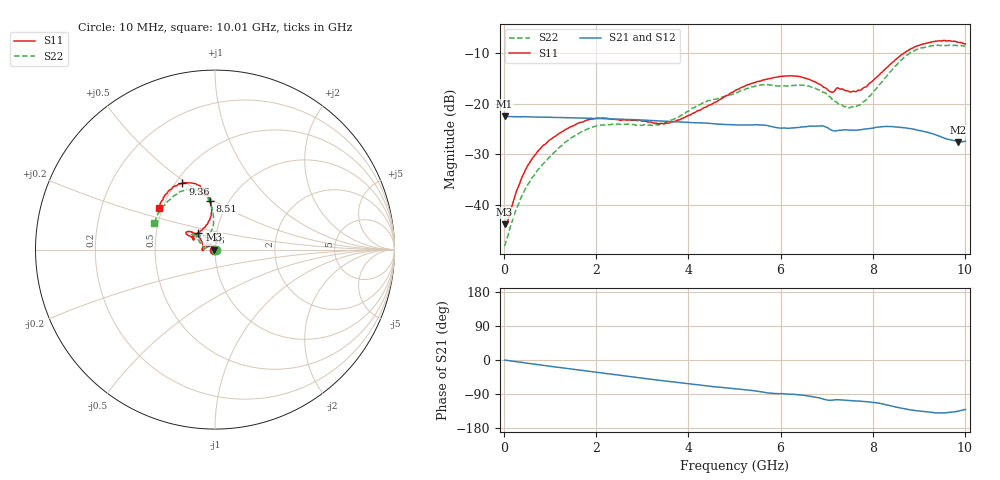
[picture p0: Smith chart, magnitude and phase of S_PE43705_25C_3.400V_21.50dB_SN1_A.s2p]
! Device ID: PE43705
! Serial: 1
! Insertion: A
! Impedance: 50 ohm
! Temp: 25C
! VDD: 3.400V
! Attenuation Step: 21.50dB
#  Hz  S  RI  R  50
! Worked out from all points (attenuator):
!   401 points, 10 MHz to 10.01 GHz, reference 50 ohm
!   highest |S21| = -22.55 dB at 10 MHz (marker M1); lowest = -27.6 dB at 9.86 GHz (marker M2)
!   lowest |S11| = -43.8 dB at 10 MHz (marker M3), VSWR 1.01, Z = 49.4 + j0.0446 ohm
!   |S11| at or under -10 dB: start of sweep to 8.683 GHz
!   |S22| runs from -48.2 to -8.5 dB; largest |S21 - S12| = 0.00085
!   S11 on the Smith chart (normalised r, x): 10 MHz: 0.99, +0.00; 7.46 GHz: 0.81, +0.16; 8.51 GHz: 0.82, +0.48; 9.36 GHz: 0.54, +0.48; 10.01 GHz: 0.48, +0.26
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1e7  -0.00643 0.000452  0.0746 -0.000322  0.0748 -0.000277  0.0039 0.000332
8.5e7  -0.00617 0.00348  0.0744 -0.00196  0.0744 -0.00195  0.00426 0.00266
3.85e8  -0.0101 0.0156  0.0735 -0.00808  0.0738 -0.00812  0.000149 0.0123
6.6e8  -0.0194 0.0236  0.0724 -0.0141  0.0724 -0.014  -0.0085 0.0178
1.035e9  -0.0365 0.0264  0.0699 -0.0216  0.0699 -0.0214  -0.025 0.0187
1.685e9  -0.0635 0.0161  0.0639 -0.033  0.0638 -0.033  -0.0522 0.00853
2.185e9  -0.0717 0.00178  0.0578 -0.0409  0.0579 -0.0409  -0.0614 -0.00153
3.36e9  -0.0633 0.00248  0.0402 -0.0542  0.0402 -0.0541  -0.0614 0.0084
3.86e9  -0.0666 0.0251  0.0321 -0.0572  0.0321 -0.0573  -0.0727 0.0266
5.01e9  -0.1039 0.0852  0.0152 -0.0598  0.0152 -0.0598  -0.1042 0.0729
5.535e9  -0.1337 0.098  0.00724 -0.0611  0.00732 -0.0611  -0.1219 0.0896
6.01e9  -0.1569 0.0991  0.00103 -0.0572  0.00126 -0.0572  -0.1199 0.0892
6.685e9  -0.1483 0.0785  -0.007 -0.0595  -0.00706 -0.0594  -0.1196 0.0809
7.085e9  -0.1152 0.0612  -0.0154 -0.0531  -0.0154 -0.0531  -0.0841 0.079
7.46e9  -0.0945 0.0942  -0.0158 -0.0524  -0.0158 -0.0524  -0.0471 0.08
7.785e9  -0.0517 0.1318  -0.0184 -0.0526  -0.0178 -0.0526  -0.0228 0.101
8.36e9  -0.0185 0.239  -0.0299 -0.0515  -0.0299 -0.0517  -0.0118 0.2017
8.51e9  -0.0275 0.2734  -0.0333 -0.0482  -0.0331 -0.0486  -0.0205 0.2378
8.91e9  -0.0818 0.3534  -0.0381 -0.0405  -0.0377 -0.0408  -0.0829 0.3249
9.36e9  -0.1818 0.3684  -0.0376 -0.0319  -0.0373 -0.0324  -0.1808 0.3265
9.86e9  -0.2895 0.2776  -0.0295 -0.0296  -0.0294 -0.0298  -0.3074 0.212
1.001e10  -0.3142 0.2298  -0.0276 -0.0323  -0.0279 -0.0324  -0.341 0.1504
